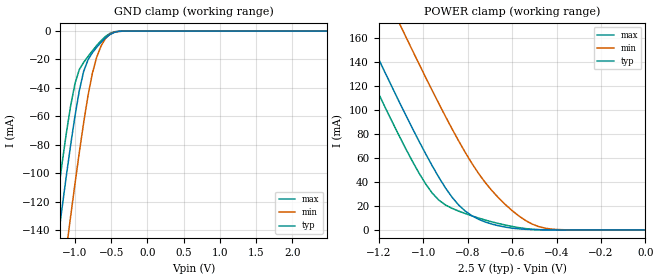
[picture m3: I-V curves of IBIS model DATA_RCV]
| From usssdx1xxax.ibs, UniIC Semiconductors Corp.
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|   Model DATA_RCV
[Model]  DATA_RCV
Model_type Input
Polarity   Non-Inverting
Vinl =   940.000mV
Vinh =   1.560V
C_comp   2.2640pF   2.2480pF   2.2810pF
[Temperature Range]   25.0000   0.1250k   -55.0000
[Voltage Range]   2.5000V   2.3000V   2.7000V
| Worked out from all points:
|   GND clamp passes 1 mA (typ) near -0.46 V on its own axis
|   POWER clamp passes 1 mA (typ) near -0.57 V on its own axis
[GND_clamp]
|Voltage   I(typ)   I(min)   I(max)
-2.5V     -683.1mA   -736.1mA   -653.6mA
-1.3V     -173.1mA   -226.8mA   -141.1mA
-1.24V    -149mA     -202.4mA   -117.2mA
-1.18V    -125.4mA   -178.1mA   -94.12mA
-1.12V    -102.4mA   -154.2mA   -72.32mA
-1.06V    -80.41mA   -130.7mA   -52.79mA
-1V       -59.95mA   -107.7mA   -37.03mA
-880mV    -28.39mA   -64.58mA   -22.05mA
-760mV    -15.32mA   -29.84mA   -13.95mA
-700mV    -11.37mA   -18.38mA   -10.19mA
-520mV    -2.567mA   -2.292mA   -1.702mA
2.48V     19.82nA    1.016uA    2.464nA
[POWER_clamp]
|Voltage   I(typ)   I(min)   I(max)
-2.49V    671mA      736.6mA    644.5mA
-1.35V    201.6mA    268.3mA    172.7mA
-1.32V    189.6mA    256.3mA    160.6mA
-1.26V    165.8mA    232.4mA    136.8mA
-1.11V    107.6mA    173.4mA    79.15mA
-1.08V    96.37mA    161.8mA    68.24mA
-960mV    53.65mA    116.5mA    30.86mA
-840mV    20.7mA     74.06mA    15.7mA
-720mV    6.602mA    39.33mA    8.242mA
-600mV    1.533mA    16.16mA    2.964mA
-450mV    76.58uA    1.436mA    135uA
0V        21.05nA    42.84nA    5.083nA
